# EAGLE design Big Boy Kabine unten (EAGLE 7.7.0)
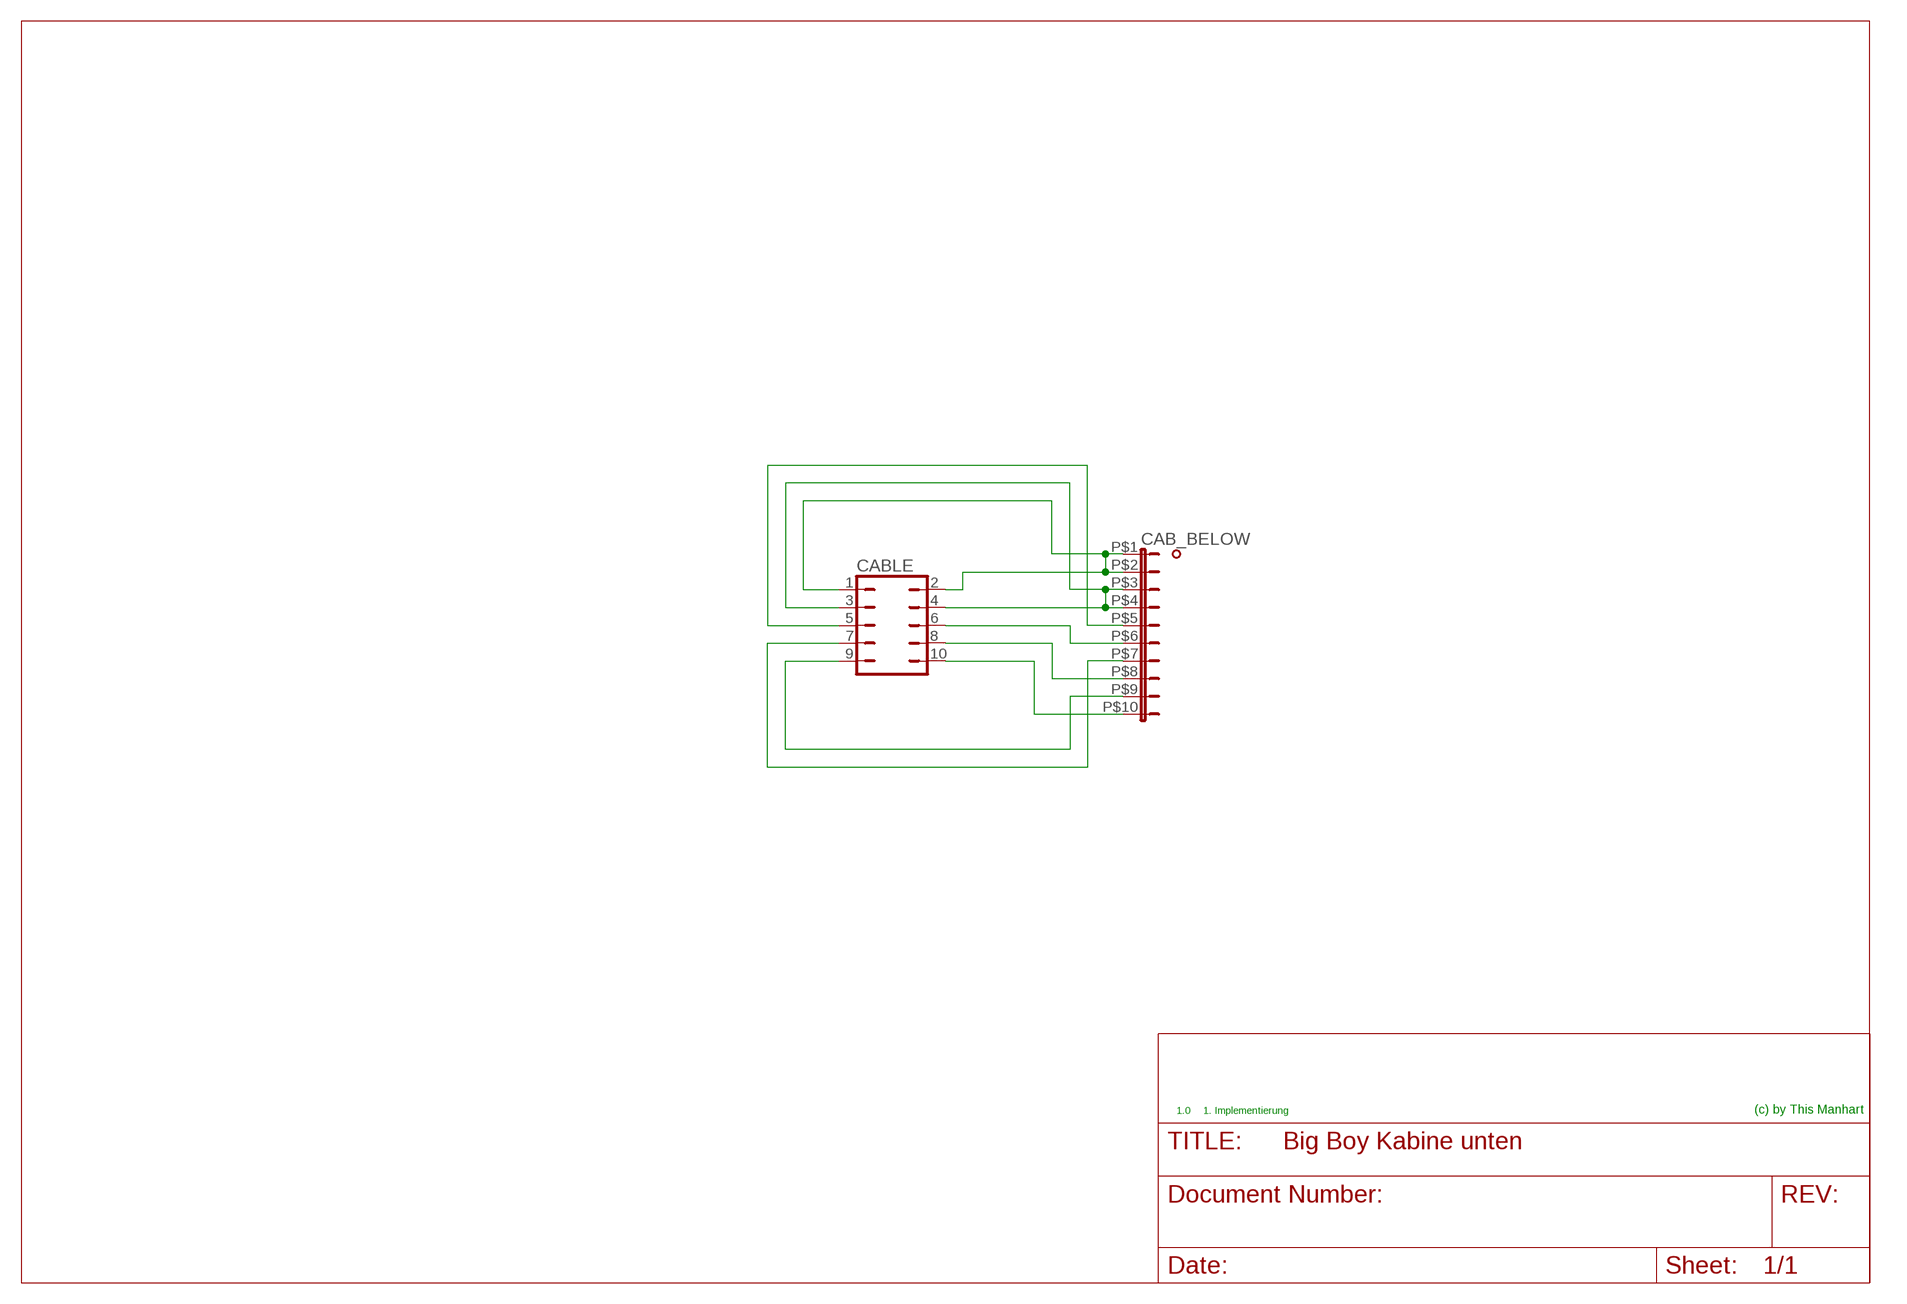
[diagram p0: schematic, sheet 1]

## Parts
CAB_BELOW  DUBOX_10POL2R_90  [DUBOX_10POL_STIFTLEISTE_90_2R]
CABLE  JUMPER_10POHNE  [JUMPER_10P_2.54_OHNE]

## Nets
N$1: CAB_BELOW.P$1 CAB_BELOW.P$2 CABLE.1 CABLE.2
N$3: CAB_BELOW.P$3 CAB_BELOW.P$4 CABLE.3 CABLE.4
N$5: CAB_BELOW.P$5 CABLE.5
N$6: CAB_BELOW.P$6 CABLE.6
N$7: CAB_BELOW.P$7 CABLE.7
N$8: CAB_BELOW.P$8 CABLE.8
N$9: CAB_BELOW.P$9 CABLE.9
N$10: CAB_BELOW.P$10 CABLE.10

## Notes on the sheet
- 1.0 | 1. Implementierung | (c) by This Manhart

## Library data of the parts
CAB_BELOW = 0_mm:DUBOX_10POL
CABLE = 0_mm:JUMPER_10P

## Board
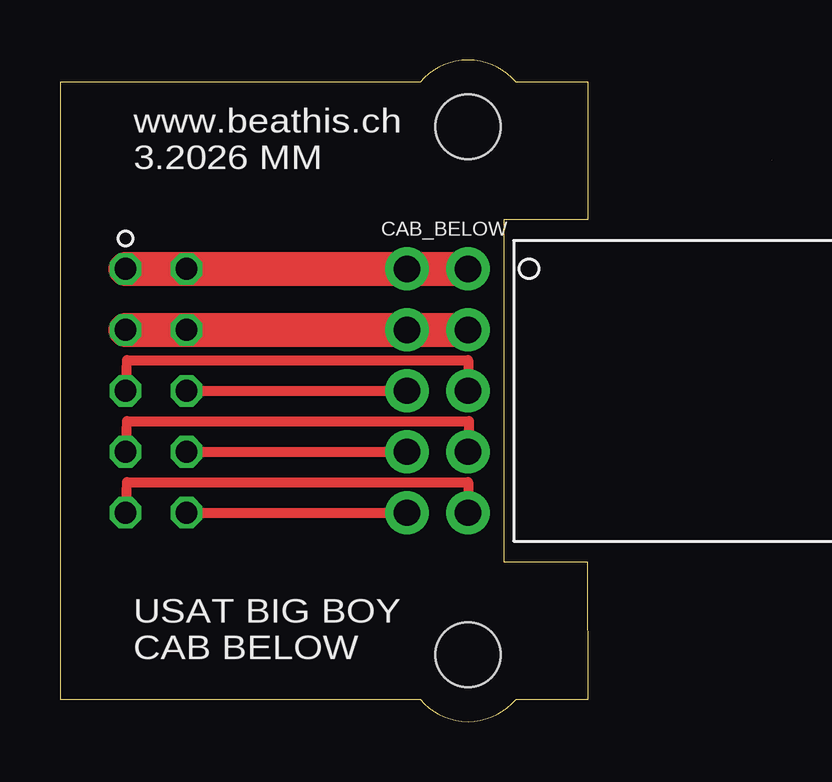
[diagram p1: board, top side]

Size 29.66 x 27.57 mm. Coordinates in mm from the lower left corner, seen from the top.
Outline: 29.65,23.38 29.66,23.38
Outline: 22,0.93 21.99,6.63 18.5,6.63 18.5,20.93 22,20.93 22,26.63 19,26.63 arc100 15,26.63 0,26.63 0,0.93 15,0.93 arc100 19,0.93 22,0.93
Copper layers (1*16): Top 0.035mm / dielectric 1.5mm / Bottom 0.035mm
Design rules "PCB-POOL Standard": minimum track width 0.15mm, minimum drill 0.3mm, track to track 0.15mm, track to pad 0.15mm, pad to pad 0.15mm, via to via 0.15mm, smd to smd 0.15mm, copper to edge 0.3mm, drill to drill 0.2mm, minimum pad ring 0.2mm, minimum via ring 0.15mm, stop-mask expansion 0.075mm, vias tented up to drill 0mil, thermal gap 0.2mm
Holes 2.7 mm at 17,2.78 17,24.78

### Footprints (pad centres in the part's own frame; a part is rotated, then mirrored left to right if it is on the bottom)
DUBOX_10POL_STIFTLEISTE_90_2R = drill 1.1 pad 1.8: P$1 -1.27,0; P$2 -1.27,-2.54; P$3 1.27,0; P$4 1.27,-2.54; P$5 3.81,0; P$6 3.81,-2.54; P$7 6.35,0; P$8 6.35,-2.54; P$9 8.89,0; P$10 8.89,-2.54
JUMPER_10P_2.54_OHNE = drill 0.914 octagon: 1 -5.08,-1.27; 2 -5.08,1.27; 3 -2.54,-1.27; 4 -2.54,1.27; 5 0,-1.27; 6 0,1.27; 7 2.54,-1.27; 8 2.54,1.27; 9 5.08,-1.27; 10 5.08,1.27

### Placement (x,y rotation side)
CAB_BELOW  17,17.59 270 top
CABLE  4,13.78 270 top

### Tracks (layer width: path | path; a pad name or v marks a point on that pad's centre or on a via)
N$1
  Top 1.422: CABLE.1 CABLE.2 CAB_BELOW.P$2 CAB_BELOW.P$1
N$3
  Top 1.422: CABLE.3 CABLE.4 CAB_BELOW.P$4 CAB_BELOW.P$3
N$5
  Top 0.406: CABLE.5 2.8,15.06 17,15.06 CAB_BELOW.P$5
N$6
  Top 0.406: CABLE.6 CAB_BELOW.P$6
N$7
  Top 0.406: CABLE.7 2.8,12.52 17.04,12.52 17.04,11.24 CAB_BELOW.P$7
N$8
  Top 0.406: CABLE.8 CAB_BELOW.P$8
N$9
  Top 0.406: CABLE.9 2.8,9.97 17,9.97 CAB_BELOW.P$9
N$10
  Top 0.406: CABLE.10 CAB_BELOW.P$10

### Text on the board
tNames: www.beathis.ch / 3.2026 MM | USAT BIG BOY / CAB BELOW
